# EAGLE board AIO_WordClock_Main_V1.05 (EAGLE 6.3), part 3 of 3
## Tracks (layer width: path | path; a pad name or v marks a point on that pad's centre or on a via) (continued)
V+  (via drill 0.5) (continued)
  Top 0.61: 73.64,139.16 45.57,139.16 | 101.7,139.16 73.64,139.16 | 129.77,139.16 101.7,139.16 | 157.96,139.16 163.42,139.16 C401.1 166.59,138 v166.6,138.02 v167.62,138.02 v168.63,138.02 | 157.96,139.16 129.77,139.16 | 186.03,139.16 178.62,139.16 C402.1 175.5,138 v175.49,138.02 v174.47,138.02 v173.46,138.02 | R405.1 129.75,139.14 129.77,139.16 | R404.1 101.65,139.11 101.7,139.16 | R403.1 73.55,139.07 73.64,139.16 | R402.1 45.45,139.04 45.57,139.16 | 15.64,91.53 R414.2 | 15.64,91.53 43.79,91.53 | 43.79,91.53 71.86,91.53 | 71.86,91.53 100.18,91.53 | 100.18,91.53 128.12,91.53 | 128.12,91.53 156.06,91.53 | 156.06,91.53 164.01,91.53 C405.1 164.52,92.04 v166.6,92.04 v167.62,92.04 v168.63,92.04 | R418.2 128.05,91.53 128.12,91.53 | R417.2 99.95,91.53 100.18,91.53 | R415.2 43.75,91.58 43.79,91.53 | R416.2 71.85,91.54 71.86,91.53 | 268.58,91.41 295.16,91.41 R424.2 | 240.39,91.41 268.58,91.41 | 212.45,91.41 240.39,91.41 | 184.13,91.41 212.45,91.41 | 184.13,91.41 178.28,91.41 C406.1 177.64,92.04 v175.49,92.04 v174.47,92.04 v173.46,92.04 | R423.2 268.55,91.44 268.58,91.41 | R422.2 240.45,91.47 240.39,91.41 | R421.2 212.35,91.5 212.45,91.41 | R420.2 184.25,91.53 184.13,91.41 | R511.1 298.35,76.35 298.35,77.16 | 270.11,77.16 298.35,77.16 | 242.29,77.16 270.11,77.16 | 214.1,77.16 242.29,77.16 | 186.03,77.16 214.1,77.16 | R510.1 270.25,77.02 270.11,77.16 | R509.1 242.15,77.02 242.29,77.16 | R508.1 214.05,77.11 214.1,77.16 | R507.1 185.95,77.08 186.03,77.16 | R501.1 18.61,77.16 45.57,77.16 | 73.64,77.16 45.57,77.16 | 101.7,77.16 73.64,77.16 | 129.77,77.16 101.7,77.16 | 157.84,77.16 163.42,77.16 C501.1 166.59,76 v166.6,76.02 v167.62,76.02 v168.63,76.02
  Top 0.61: 157.84,77.16 129.77,77.16 | 186.03,77.16 178.62,77.16 C502.1 175.5,76 v175.49,76.02 v174.47,76.02 v173.46,76.02 | R505.1 129.75,77.14 129.77,77.16 | R504.1 101.65,77.11 101.7,77.16 | R503.1 73.55,77.07 73.64,77.16 | R502.1 45.45,77.04 45.57,77.16 | R514.2 17.02,29.53 43.79,29.53 | 71.86,29.53 43.79,29.53 | 100.18,29.53 71.86,29.53 | 128.12,29.53 100.18,29.53 | 156.19,29.53 164.01,29.53 C505.1 164.52,30.04 v166.6,30.04 v167.62,30.04 v168.63,30.04 | 156.19,29.53 128.12,29.53 | R518.2 128.05,29.53 128.12,29.53 | R517.2 99.95,29.53 100.18,29.53 | R515.2 43.75,29.58 43.79,29.53 | R516.2 71.85,29.54 71.86,29.53 | 268.58,29.41 295.16,29.41 R524.2 | 240.39,29.41 268.58,29.41 | 212.45,29.41 240.39,29.41 | 184.13,29.41 212.45,29.41 | 184.13,29.41 178.28,29.41 C506.1 177.64,30.04 v175.49,30.04 v174.47,30.04 v173.46,30.04 | R523.2 268.55,29.44 268.58,29.41 | R522.2 240.45,29.47 240.39,29.41 | R521.2 212.35,29.5 212.45,29.41 | R520.2 184.25,29.53 184.13,29.41 | 15.64,91.53 9.18,91.53 7.6,89.96 7.6,27.6 9.63,25.57 9.63,13.5 8.61,12.49 J401A.3 J401A.1 J401.1 J401.3 | 298.35,77.16 308.71,77.16 310.13,75.73 310.13,28.64 306.3,24.8 J501.3 J501.1 J501A.1 J501A.3 | R106.1 157.85,325.05 157.96,325.16 | R119.2 156.15,277.57 156.19,277.53 | R206.1 157.84,261.9 157.84,263.16 | R219.2 156.19,216.9 156.19,215.53 | R319.2 156.15,153.63 156.06,153.53 | R306.1 157.85,201.15 157.84,201.16 | R406.1 157.96,137.9 157.96,139.16 | R419.2 156.15,91.63 156.06,91.53 | R506.1 157.85,77.15 157.84,77.16 | R519.2 156.15,29.57 156.19,29.53 | U601.7 278.48,6.38 278.36,6.26
  Top 1.27: v173.08,26.71 v174.09,26.71 v175.11,26.71 v176.12,26.71 v177.14,26.71 300.08,26.71 302.62,24.17 302.62,7.41 299.82,4.61 283.06,4.61 C604.1 C615.1 278.36,6.26
  Bottom 1.27: v166.6,324.02 v167.62,324.02 v168.63,324.02 171.68,324.02 | 171.68,324.02 v173.46,324.02 v174.47,324.02 v175.49,324.02 | v166.6,278.04 v167.62,278.04 v168.63,278.04 171.68,278.04 | 171.68,278.04 v173.46,278.04 v174.47,278.04 v175.49,278.04 | v166.6,262.02 v167.62,262.02 v168.63,262.02 171.68,262.02 | 171.68,262.02 v173.46,262.02 v174.47,262.02 v175.49,262.02 | v166.6,216.04 v167.62,216.04 v168.63,216.04 171.68,216.04 | 171.68,216.04 v173.46,216.04 v174.47,216.04 v175.49,216.04 | v166.6,200.02 v167.62,200.02 v168.63,200.02 171.68,200.02 | 171.68,200.02 v173.33,200.02 v174.35,200.02 v175.36,200.02 | v166.6,154.04 v167.62,154.04 v168.63,154.04 171.68,154.04 | 171.68,154.04 v173.46,154.04 v174.47,154.04 v175.49,154.04 | v166.6,138.02 v167.62,138.02 v168.63,138.02 171.68,138.02 | 171.68,138.02 v173.46,138.02 v174.47,138.02 v175.49,138.02 | v166.6,92.04 v167.62,92.04 v168.63,92.04 171.68,92.04 | 171.68,92.04 v173.46,92.04 v174.47,92.04 v175.49,92.04 | v166.6,76.02 v167.62,76.02 v168.63,76.02 171.68,76.02 | 171.68,76.02 v173.46,76.02 v174.47,76.02 v175.49,76.02 | v166.6,30.04 v167.62,30.04 v168.63,30.04 171.68,30.04 | 171.68,30.04 v173.46,30.04 v174.47,30.04 v175.49,30.04 | 171.68,278.04 171.68,295.95 175.49,299.76 175.49,302.94 171.68,306.75 171.68,324.02 | 171.68,262.02 171.68,278.04 | 171.68,216.04 171.68,262.02 | 171.68,200.02 171.68,216.04 | 171.68,154.04 171.68,171.49 175.49,175.3 175.49,179.11 171.68,182.92 171.68,200.02 | 171.68,138.02 171.68,154.04 | 171.68,92.04 171.68,138.02 | 171.68,92.04 171.68,76.02 | 171.68,76.02 171.68,59.73 175.49,55.92 175.49,50.84 171.68,47.03 171.68,30.04
  Bottom 1.27: 171.68,30.04 171.68,28.11 v173.08,26.71 v174.09,26.71 v175.11,26.71 v176.12,26.71 v177.14,26.71

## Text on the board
Top: TOP | TOP | TOP
Bottom: BOT | BOT | BOT
tPlace: E | S | K | I | S | T | L | F | Ü | N | F | Z | E | H | N | Z | W | A | N | Z | I | G | D | R | E | I | V | I | E | R | T | E | L | T | G | N | A | C | H | V | O | R | J | M | H | A | L | B | Q | Z | W | Ö | L | F | P | Z | W | E | I | N | S | I | E | B | E | N | K | D | R | E | I | R | H | F | Ü | N | F | E | L | F | N | E | U | N | V | I | E | R | W | A | C | H | T | Z | E | H | N | R | S | B | S | E | C | H | S | F | M | U | H | R | tPL | DCF-77 Receiver | Minute | Bottom | Bottom | LEDs | Left | Right | Right | 3 | 4 | 3 | 4 | LCD + Keyboard | Minute | USB & Power | DCF-77 | LEDs | 1 | 2 | 1 | 2 | Top | Top | Rcv. | Left | tPL | tPL | Left | Right
bPlace: DCF-77 | Rcv. | PA3 | PA4 | PA5 | PA6 | PE7 | PE6 | PA7 | PB0 | PE5 | PE4 | PE3 | PE2 | PB4 | PB5 | PE1 | PB6 | PE0 | PB7 | +3V3 | bPl | Minute | GND | LEDs | Right | Minute | LEDs | Left | bPl | bPl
